|Texas Instruments Incorporated
| IBIS Model of : TMUX6219
| 38V 2:1 Analog Multiplexer
| This file contains package information for the following:
|  VSSOP 8-pin (DGK) package as [Component] TMUX6219_DGK
|  WSON  8-pin (RQX) package as [Component] TMUX6219_RQX
| This device can be powered at the following Vccs:
| Single Rail Supply Configurations:
|  5.0 volt VDD, 0V VSS
|  12.0 volt VDD, 0V VSS
|  36.0 volt VDD, 0V VSS
| Dual Rail Supply Configurations:
|  5.0 volt VDD, -5V VSS
|  15.0 volt VDD, -15V VSS
| Digital Voltage Range : 4.5-38
| Package-type: VSSOP 8-pin
| #pins/pkg drawing : 8-pin DGK
[IBIS Ver] 4.1
[File name] TMUX6219.ibs
[File Rev] 1.2
[Date] 07/19/2022
[Source]
| Texas Instruments Incorporated.
| 12500 TI Blvd
| Dallas, TX -75243
[Notes] Revision History:
| Rev 1.0: 09/03/2020
| - Initial version of the model
| - Model generated from simulations in TISPICE/SPECTRE
| - C_comp although listed in numerical order of value are
| obtained from varying PVT conditions. For PVT conditions for
| each specific value refer the buffer description under
| respective [Model]. IBIS model user is responsible for using
| appropriate C_comp to simulate for Signal Integrity.
| - Warnings regarding combined Non-monotonicity of various models have been
| reviewed and considered minor and can be ignored.
| Rev 1.1: 01/06/2021
| - Updated Off Leakage Current
| Rev 1.2: 05/03/2022
| - Added RQX package
|**** Modify the following if you use [Model Selector]***********
| - Model names with a trailing voltage extension contain the model for
| operation at that voltage range.
[Disclaimer]
| This model is designed as an aid for customers of Texas Instruments.
| TI and its licensors and suppliers make no warranties, either expressed
| or implied, with respect to this model, including the warranties of
| merchantability or fitness for a particular purpose. The model is
| provided solely on an "as is" basis. The entire risk as to its quality
| and performance is with the customer.
| This model is subject to change without notice. Texas Instruments
| Incorporated is not responsible for updating this model.
[Copyright]
(C) Copyright 2022 Texas Instruments Incorporated. All rights reserved.
| Component TMUX6219_DGK 8-pin SOT (per package)
[Component] TMUX6219_DGK
[Manufacturer]  Texas Instruments Incorporated
[Package] |VSSOP (DGK) 8-pin
| variable typ min max
R_pkg 0.05 0.04 0.06
L_pkg 1.0nH 0.8nH 1.2nH
C_pkg 0.2pF 0.16pF 0.24pF
| pin number (pin name) mapping to model name
[Pin] signal_name   model_name   R_pin L_pin C_pin
1   D   TMUX6219_DX   NA   NA   NA
2   SA   TMUX6219_SX   NA   NA   NA
3   GND   GND   NA   NA   NA
4   VDD   POWER   NA   NA   NA
5   EN   INPUT_PU   NA   NA   NA
6   IN   INPUT_PD   NA   NA   NA
7   VSS   POWER   NA   NA   NA
8   SB   TMUX6219_SX   NA   NA   NA
[Series Switch Groups]
| Function Group States
On  1 /   | SB->D IN HIGH  EN HIGH
   | D->SB IN HIGH  EN HIGH
On  2 /   | SA->D IN LOW   EN HIGH
   | D->SA IN LOW   EN HIGH
Off 1 2 /   | EN LOW
[Series Pin Mapping]   pin_2   model_name   function_table_group
8   1   TMUX6219_SX_SINGLE_5V_S   1
1   8   TMUX6219_DX_SINGLE_5V_S   1
2   1   TMUX6219_SX_SINGLE_5V_S   2
1   2   TMUX6219_DX_SINGLE_5V_S   2
| 8   1   TMUX6219_SX_SINGLE_12V_S   1
| 1   8   TMUX6219_DX_SINGLE_12V_S   1
| 2   1   TMUX6219_SX_SINGLE_12V_S   2
| 1   2   TMUX6219_DX_SINGLE_12V_S   2
| 8   1   TMUX6219_SX_SINGLE_36V_S   1
| 1   8   TMUX6219_DX_SINGLE_36V_S   1
| 2   1   TMUX6219_SX_SINGLE_36V_S   2
| 1   2   TMUX6219_DX_SINGLE_36V_S   2
| 8   1   TMUX6219_SX_SINGLE_36V_S   1
| 1   8   TMUX6219_DX_SINGLE_36V_S   1
| 2   1   TMUX6219_SX_SINGLE_36V_S   2
| 1   2   TMUX6219_DX_SINGLE_36V_S   2
| 8   1   TMUX6219_SX_DUAL_PM5_S   1
| 1   8   TMUX6219_DX_DUAL_PM5_S   1
| 2   1   TMUX6219_SX_DUAL_PM5_S   2
| 1   2   TMUX6219_DX_DUAL_PM5_S   2
| 8   1   TMUX6219_SX_DUAL_PM15_S   1
| 1   8   TMUX6219_DX_DUAL_PM15_S   1
| 2   1   TMUX6219_SX_DUAL_PM15_S   2
| 1   2   TMUX6219_DX_DUAL_PM15_S   2
| Component TMUX6219_RQX 8-pin SOT (per package)
[Component] TMUX6219_RQX
[Manufacturer]  Texas Instruments Incorporated
[Package] |WSON (RQX) 8-pin
| variable typ min max
R_pkg 0.05 0.04 0.06
L_pkg 1.0nH 0.8nH 1.2nH
C_pkg 0.2pF 0.16pF 0.24pF
| pin number (pin name) mapping to model name
[Pin] signal_name   model_name   R_pin L_pin C_pin
1   D   TMUX6219_DX   NA   NA   NA
2   SA   TMUX6219_SX   NA   NA   NA
3   GND   GND   NA   NA   NA
4   VDD   POWER   NA   NA   NA
5   EN   INPUT_PU   NA   NA   NA
6   IN   INPUT_PD   NA   NA   NA
7   VSS   POWER   NA   NA   NA
8   SB   TMUX6219_SX   NA   NA   NA
[Series Switch Groups]
| Function Group States
|On  1 /   | SB->D IN HIGH  EN HIGH
|   | D->SB IN HIGH  EN HIGH
|On  2 /   | SA->D IN LOW   EN HIGH
|   | D->SA IN LOW   EN HIGH
|Off 1 2 /   | EN LOW
[Series Pin Mapping]   pin_2   model_name   function_table_group
| 8   1   TMUX6219_SX_SINGLE_5V_S   1
| 1   8   TMUX6219_DX_SINGLE_5V_S   1
| 2   1   TMUX6219_SX_SINGLE_5V_S   2
| 1   2   TMUX6219_DX_SINGLE_5V_S   2
| 8   1   TMUX6219_SX_SINGLE_12V_S   1
| 1   8   TMUX6219_DX_SINGLE_12V_S   1
| 2   1   TMUX6219_SX_SINGLE_12V_S   2
| 1   2   TMUX6219_DX_SINGLE_12V_S   2
 8   1   TMUX6219_SX_SINGLE_36V_S   1
 1   8   TMUX6219_DX_SINGLE_36V_S   1
 2   1   TMUX6219_SX_SINGLE_36V_S   2
 1   2   TMUX6219_DX_SINGLE_36V_S   2
| 8   1   TMUX6219_SX_DUAL_PM5_S   1
| 1   8   TMUX6219_DX_DUAL_PM5_S   1
| 2   1   TMUX6219_SX_DUAL_PM5_S   2
| 1   2   TMUX6219_DX_DUAL_PM5_S   2
| 8   1   TMUX6219_SX_DUAL_PM15_S   1
| 1   8   TMUX6219_DX_DUAL_PM15_S   1
| 2   1   TMUX6219_SX_DUAL_PM15_S   2
| 1   2   TMUX6219_DX_DUAL_PM15_S   2
| Model Selectors
|*** power supply options or driver programmability *********
[Model Selector] INPUT_PU
INBUF_PU_5V   INPUT_PU   buffer at 5V operation.
INBUF_PU_12V   INPUT_PU   buffer at 12V operation.
INBUF_PU_15V   INPUT_PU   buffer at 15V operation.
INBUF_PU_20V   INPUT_PU   buffer at 20V operation.
INBUF_PU_36V   INPUT_PU   buffer at 36V operation.
[Model Selector] INPUT_PD
INBUF_PD_5V   INPUT_PD   buffer at 5V operation.
INBUF_PD_12V   INPUT_PD   buffer at 12V operation.
INBUF_PD_15V   INPUT_PD   buffer at 15V operation.
INBUF_PD_20V   INPUT_PD   buffer at 20V operation.
INBUF_PD_36V   INPUT_PD   buffer at 36V operation.
[Model Selector] TMUX6219_SX
TMUX6219_SX_SINGLE_5V  switch termination at +5V operation.
TMUX6219_SX_SINGLE_12V  switch termination at +12V operation.
TMUX6219_SX_SINGLE_36V  switch termination at +36V operation.
TMUX6219_SX_DUAL_PM5  switch termination at +/-5V operation.
TMUX6219_SX_DUAL_PM15  switch termination at +/-15V operation.
[Model Selector] TMUX6219_SX_S
TMUX6219_SX_SINGLE_5V_S  switch at +5V operation.
TMUX6219_SX_SINGLE_12V_S  switch at +12V operation.
TMUX6219_SX_SINGLE_36V_S  switch at +36V operation.
TMUX6219_SX_DUAL_PM5_S  switch at +/-5V operation.
TMUX6219_SX_DUAL_PM15_S  switch at +/-15V operation.
[Model Selector] TMUX6219_DX
TMUX6219_DX_SINGLE_5V  termination switch at +5V operation.
TMUX6219_DX_SINGLE_12V  termination switch at +12V operation.
TMUX6219_DX_SINGLE_36V  termination switch at +36V operation.
TMUX6219_DX_DUAL_PM5  termination switch at +/-5V operation.
TMUX6219_DX_DUAL_PM15  termination switch at +/-15V operation.
[Model Selector] TMUX6219_DX_S
TMUX6219_DX_SINGLE_5V_S  switch at +5V operation.
TMUX6219_DX_SINGLE_12V_S  switch at +12V operation.
TMUX6219_DX_SINGLE_36V_S  switch at +36V operation.
TMUX6219_DX_DUAL_PM5_S  switch at +/-5V operation.
TMUX6219_DX_DUAL_PM15_S  switch at +/-15V operation.
[Model]   TMUX6219_SX_SINGLE_5V_S
Model_type  Series_switch
| variable   typ   min   max
C_comp   110pF   110pF   110pF
[Temperature Range]   25   125   -40
| Ambient temperature   25   125   -40
[Voltage range]   5   5   5
[On]
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[Off]
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[Model]   TMUX6219_DX_SINGLE_5V_S
Model_type  Series_switch
| variable   typ   min   max
C_comp   110pF   110pF   110pF
[Temperature Range]   25   125   -40
| Ambient temperature   25   125   -40
[Voltage range]   5   5   5
[On]
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[Off]
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[Model]   TMUX6219_SX_SINGLE_12V_S
Model_type  Series_switch
| variable   typ   min   max
C_comp   155pF   155pF   155pF
[Temperature Range]   25   125   -40
| Ambient temperature   25   125   -40
[Voltage range]   12   12   12
[On]
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[Off]
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[Model]   TMUX6219_DX_SINGLE_12V_S
Model_type  Series_switch
| variable   typ   min   max
C_comp   155pF   155pF   155pF
[Temperature Range]   25   125   -40
| Ambient temperature   25   125   -40
[Voltage range]   12   12   12
[On]
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[Off]
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[Model]   TMUX6219_SX_SINGLE_36V_S
Model_type  Series_switch
| variable   typ   min   max
C_comp   148pF   148pF   148pF
[Temperature Range]   25   125   -40
| Ambient temperature   25   125   -40
[Voltage range]   36   36   36
[On]
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[Off]
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[Model]   TMUX6219_DX_SINGLE_36V_S
Model_type  Series_switch
| variable   typ   min   max
C_comp   148pF   148pF   148pF
[Temperature Range]   25   125   -40
| Ambient temperature   25   125   -40
[Voltage range]   36   36   36
[On]
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[Off]
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[Model]   TMUX6219_SX_DUAL_PM5_S
Model_type  Series_switch
| variable   typ   min   max
C_comp   120pF   120pF   120pF
[Temperature Range]   25   125   -40
| Ambient temperature   25   125   -40
[Voltage range]   0   -5   5
[On]
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[Off]
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[Model]   TMUX6219_DX_DUAL_PM5_S
Model_type  Series_switch
| variable   typ   min   max
C_comp   120pF   120pF   120pF
[Temperature Range]   25   125   -40
| Ambient temperature   25   125   -40
[Voltage range]   0   -5   5
[On]
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[Off]
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[Model]   TMUX6219_SX_DUAL_PM15_S
Model_type  Series_switch
| variable   typ   min   max
C_comp   150pF   150pF   150pF
[Temperature Range]   25   125   -40
| Ambient temperature   25   125   -40
[Voltage range]   0   -15   15
[On]
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[Off]
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[Model]   TMUX6219_DX_DUAL_PM15_S
Model_type  Series_switch
| variable   typ   min   max
C_comp   150pF   150pF   150pF
[Temperature Range]   25   125   -40
| Ambient temperature   25   125   -40
[Voltage range]   0   -15   15
[On]
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[Off]
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| Models and submodels in the file (30): INBUF_PD_5V (Input), INBUF_PD_12V (Input), INBUF_PD_15V (Input), INBUF_PD_20V (Input), INBUF_PD_36V (Input), INBUF_PU_5V (Input), INBUF_PU_12V (Input), INBUF_PU_15V (Input), INBUF_PU_20V (Input), INBUF_PU_36V (Input), TMUX6219_SX_SINGLE_5V_S (Series_switch), TMUX6219_SX_SINGLE_5V (Terminator), TMUX6219_DX_SINGLE_5V_S (Series_switch), TMUX6219_DX_SINGLE_5V (Terminator), TMUX6219_SX_SINGLE_12V_S (Series_switch), TMUX6219_SX_SINGLE_12V (Terminator), TMUX6219_DX_SINGLE_12V_S (Series_switch), TMUX6219_DX_SINGLE_12V (Terminator), TMUX6219_SX_SINGLE_36V_S (Series_switch), TMUX6219_SX_SINGLE_36V (Terminator), TMUX6219_DX_SINGLE_36V_S (Series_switch), TMUX6219_DX_SINGLE_36V (Terminator), TMUX6219_SX_DUAL_PM5_S (Series_switch), TMUX6219_SX_DUAL_PM5 (Terminator), TMUX6219_DX_DUAL_PM5_S (Series_switch), TMUX6219_DX_DUAL_PM5 (Terminator), TMUX6219_SX_DUAL_PM15_S (Series_switch), TMUX6219_SX_DUAL_PM15 (Terminator), TMUX6219_DX_DUAL_PM15_S (Series_switch), TMUX6219_DX_DUAL_PM15 (Terminator)
